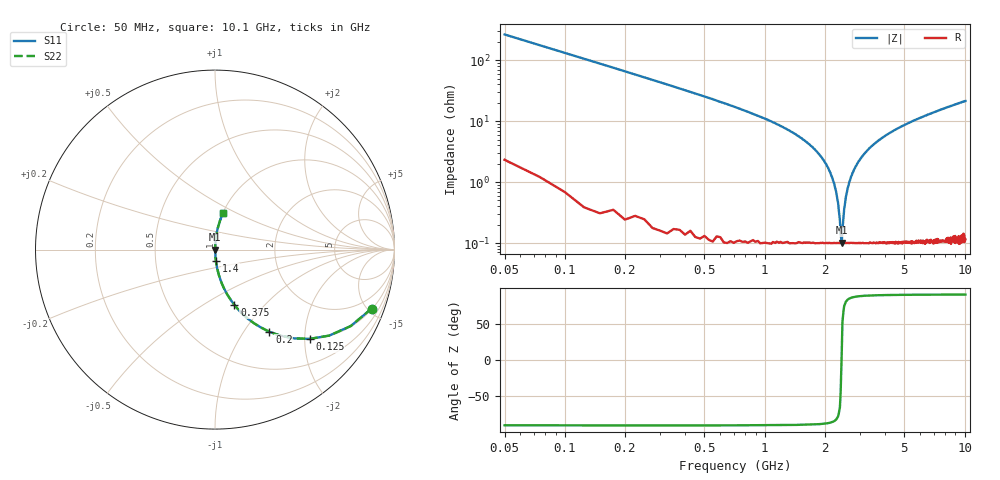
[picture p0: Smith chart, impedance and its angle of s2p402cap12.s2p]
! AVX Thin Film Operation		Date: April 2003
! Description: Accu-P® Series, Thin Film, SMD, RF Capacitor
! Part Number: 0402ZK120FBW
! 50 MHz  -  10.05 GHz
! Serial Measurements
# hz S db R 50
!	S11		S21		S12		S22
!	dB	Phase	dB	Phase	dB	Phase	dB	Phase
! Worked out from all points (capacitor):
!   400 points, 50 MHz to 10.1 GHz, reference 50 ohm
!   read as one part in series: C = 12 pF near 100 MHz
!   lowest |Z| = 101 mohm at 2.43 GHz (marker M1)
!   series resonance near 2.426 GHz, so ESL is about 360 pH
!   S11 on the Smith chart (normalised r, x): 50 MHz: 1.05, -5.30; 125 MHz: 1.01, -2.12; 200 MHz: 1.00, -1.32; 375 MHz: 1.00, -0.69; 1.4 GHz: 1.00, -0.13; 10.1 GHz: 1.00, +0.43
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5e7  -0.60 -20.6  -9.07 68.9  -9.07 68.9  -0.60 -20.6
1.25e8  -2.79 -43.3  -3.28 46.5  -3.28 46.5  -2.79 -43.3
2e8  -5.21 -56.5  -1.58 33.3  -1.58 33.3  -5.21 -56.5
3.75e8  -9.74 -70.7  -0.50 19.0  -0.50 19.0  -9.74 -70.7
7.75e8  -16.40 -80.9  -0.11 8.7  -0.11 8.7  -16.40 -80.9
1.4e9  -24.00 -85.5  -0.03 3.6  -0.03 3.6  -24.00 -85.5
1.73e9  -28.40 -86.3  -0.01 2.2  -0.01 2.2  -28.40 -86.3
2.03e9  -34.10 -86.0  -0.01 1.1  -0.01 1.1  -34.10 -86.0
2.23e9  -40.60 -83.3  -0.01 0.5  -0.01 0.5  -40.60 -83.3
2.33e9  -46.80 -77.1  -0.01 0.3  -0.01 0.3  -46.80 -77.1
2.38e9  -52.60 -64.7  -0.01 0.1  -0.01 0.1  -52.60 -64.7
2.4e9  -57.10 -44.2  -0.01 0.1  -0.01 0.1  -57.10 -44.2
2.43e9  -59.90 9.1  -0.01 -0.0  -0.01 -0.0  -59.90 9.1
2.5e9  -48.80 73.8  -0.01 -0.2  -0.01 -0.2  -48.80 73.8
2.55e9  -44.80 79.7  -0.01 -0.3  -0.01 -0.3  -44.80 79.7
2.7e9  -38.40 84.5  -0.01 -0.7  -0.01 -0.7  -38.40 84.5
2.95e9  -33.20 86.1  -0.01 -1.2  -0.01 -1.2  -33.20 86.1
3.4e9  -28.40 86.3  -0.01 -2.2  -0.01 -2.2  -28.40 86.3
5.08e9  -21.10 84.3  -0.04 -5.1  -0.04 -5.1  -21.10 84.3
6.75e9  -17.60 82.0  -0.09 -7.6  -0.09 -7.6  -17.60 82.0
8.43e9  -15.30 79.7  -0.14 -9.9  -0.14 -9.9  -15.30 79.7
1.01e10  -13.60 77.6  -0.20 -12.1  -0.20 -12.1  -13.60 77.6
